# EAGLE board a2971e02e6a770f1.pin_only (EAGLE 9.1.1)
REV: C

Size 60 x 60 mm. Coordinates in mm from the lower left corner, seen from the top.
Outline: 60,0 0,0 0,60 60,60 60,0
Copper layers (1*16): Top 0.035mm / dielectric 1.5mm / Bottom 0.035mm
Design rules "adafruit 88 *": minimum track width 8mil, minimum drill 15.5mil, track to track 8mil, track to pad 8mil, pad to pad 8mil, via to via 8mil, smd to smd 8mil, copper to edge 10mil, drill to drill 8mil, minimum pad ring 10mil, minimum via ring 8mil, stop-mask expansion 2mil, vias tented up to drill 20mil, thermal gap 10mil
Net classes: 1 power: width 0.406 mm; 2 gnd: width 0.254 mm
Holes 2.8 mm at 2.03,44.97 28.03,44.97 32.03,44.97 58.03,44.97 2.03,14.97 28.03,14.97 32.03,14.97 58.03,14.97
Holes 2 mm at 15.03,44.97 45.03,44.97 15.03,14.97 45.03,14.97
Holes 1 mm at 1.33,58.67 58.73,58.67 1.33,1.27 58.73,1.27

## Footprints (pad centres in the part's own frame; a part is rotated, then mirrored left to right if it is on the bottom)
0805-NO = smd 1.24 x 1.5: 1 -0.95,0; 2 0.95,0
0603-NO = smd 1.075 x 1: 1 -0.85,0; 2 0.85,0
SOD-323 = smd 1.35 x 0.8: A 1.27,0; C -1.27,0
FIDUCIAL_1MM = smd 1 x 1: 1 0,0
QFN24_4MM = smd 0.8 x 0.28: 1 -2,1.25; 2 -2,0.75; 3 -2,0.25; 4 -2,-0.25; 5 -2,-0.75; 6 -2,-1.25; 13 2,-1.25; 14 2,-0.75; 15 2,-0.25; 16 2,0.25; 17 2,0.75; 18 2,1.25 | smd 0.28 x 0.8: 7 -1.25,-2; 8 -0.75,-2; 9 -0.25,-2; 10 0.25,-2; 11 0.75,-2; 12 1.25,-2; 19 1.25,2; 20 0.75,2; 21 0.25,2; 22 -0.25,2; 23 -0.75,2; 24 -1.25,2 | smd 1.778 x 1.778: THERM 0,0
SOT23-5 = smd 0.69 x 0.99: 1 -0.95,-1.29; 2 0,-1.29; 3 0.95,-1.29; 4 0.95,1.3; 5 -0.95,1.3
5P_EDGECONNECT = smd 1.27 x 5.08: 1 -5.08,0; 2 -2.54,0; 3 0,0; 4 2.54,0; 5 5.08,0
LED3535 = smd 1 x 0.85: 1 -1.75,0.875; 2 -1.75,-0.875; 3 1.75,-0.875; 4 1.75,0.875
SOT23-WIDE = smd 1 x 1.2: 1 -0.95,-1; 2 0.95,-1; 3 0,1
SOLDERJUMPER_ARROW_NOPASTE = smd 0.762 x 1.524: 1 -1.016,0; 2 1.016,0
SOLDERJUMPER_2WAY_OPEN_NOPASTE = smd 1.168 x 1.6: 1 -1.397,0; 2 0,0; 3 1.397,0
TESTPOINT_SMT = smd 4.7 x 3.4: P$1 0,0
TESTPOINT_ROUND_2MM = smd 2 x 2: P$1 0,0
TESTPOINT_ROUND_1.5MM = smd 1.5 x 1.5: P$1 0,0
SOT23-5' = smd 0.55 x 1.2: 1 -0.95,-1.3; 2 0,-1.3; 3 0.95,-1.3; 4 0.95,1.3; 5 -0.95,1.3
MOUNTINGHOLE_2.5_PLATED = drill 2.5 pad 3.2: P$1 0,0
ELAST_PAD_SQUARE_10MM_4X4WIDE = smd 1.45 x 0.635: P$1 -3.4,0 | smd 0.305 x 0.61: P$2 4,0
JSTPH4 = smd 1 x 4.6: 1 -3,-3.7; 2 -1,-3.7; 3 1,-3.7; 4 3,-3.7 | smd 1.7 x 3.4: NC1 -5.7,1.5; NC2 5.7,1.5

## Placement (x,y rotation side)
C1  10u  [0805-NO]  52.13,26.04 0 top
C2  10u  [0805-NO]  8.69,26.16 270 top
C3  10u  [0805-NO]  31.55,6.1 0 top
C4  10u  [0805-NO]  33.84,52.7 90 top
C7  1uF  [0603-NO]  25.58,47.85 0 top
C8  10µF  [0805-NO]  24.63,45.22 270 top
D1  1N4148  [SOD-323]  37.59,48.95 180 top
D2  1N4148  [SOD-323]  22.59,48.95 0 top
D3  1N4148  [SOD-323]  9.66,50.09 0 top
D4  1N4148  [SOD-323]  52.62,40.96 180 top
D5  1N4148  [SOD-323]  37.61,40.96 180 top
D6  1N4148  [SOD-323]  22.69,40.96 0 top
D7  1N4148  [SOD-323]  7.92,40.71 0 top
D8  1N4148  [SOD-323]  52.68,18.97 180 top
D9  1N4148  [SOD-323]  52.58,48.94 180 top
D10  1N4148  [SOD-323]  37.7,18.84 180 top
D11  1N4148  [SOD-323]  14.06,18.86 180 top
D12  1N4148  [SOD-323]  7.4,18.83 0 top
D13  1N4148  [SOD-323]  52.48,11.01 180 top
D14  1N4148  [SOD-323]  37.62,11.01 180 top
D15  1N4148  [SOD-323]  13.11,10.98 180 top
D16  1N4148  [SOD-323]  7.45,11.02 0 top
FID1  FIDUCIAL_1MM  [FIDUCIAL_1MM]  10.23,14.05 0 top
FID2  FIDUCIAL_1MM  [FIDUCIAL_1MM]  58.48,11.68 0 top
FID3  FIDUCIAL_1MM  [FIDUCIAL_1MM]  56.25,54.98 0 top
FID4  FIDUCIAL_1MM  [FIDUCIAL_1MM]  51.36,46.1 0 bottom
FID5  FIDUCIAL_1MM  [FIDUCIAL_1MM]  44.76,7.11 0 bottom
FID6  FIDUCIAL_1MM  [FIDUCIAL_1MM]  7.93,15.75 0 bottom
IC2  ATSAMD09D14A-MU  [QFN24_4MM]  38.96,31.87 270 top
IC3  74AHCT1G125DBV  [SOT23-5]  47.3,50.29 90 top
JP1  [5P_EDGECONNECT]  2.6,29.97 90 top
JP2  [5P_EDGECONNECT]  57.46,29.97 90 top
JP3  [5P_EDGECONNECT]  30.03,2.54 180 top
JP4  [5P_EDGECONNECT]  30.03,57.4 180 top
LED1  WS2812B3535  [LED3535]  52.53,52.47 270 bottom
LED2  WS2812B3535  [LED3535]  37.53,52.47 270 bottom
LED3  WS2812B3535  [LED3535]  22.53,52.47 270 bottom
LED4  WS2812B3535  [LED3535]  7.53,52.47 270 bottom
LED5  WS2812B3535  [LED3535]  52.53,37.47 270 bottom
LED6  WS2812B3535  [LED3535]  37.53,37.47 270 bottom
LED7  WS2812B3535  [LED3535]  22.53,37.47 270 bottom
LED8  WS2812B3535  [LED3535]  7.53,37.47 270 bottom
LED9  WS2812B3535  [LED3535]  52.53,22.47 270 bottom
LED10  WS2812B3535  [LED3535]  37.53,22.47 270 bottom
LED11  WS2812B3535  [LED3535]  7.53,22.47 270 bottom
LED12  WS2812B3535  [LED3535]  22.53,22.47 270 bottom
LED13  WS2812B3535  [LED3535]  52.53,7.47 270 bottom
LED14  WS2812B3535  [LED3535]  37.53,7.47 270 bottom
LED15  WS2812B3535  [LED3535]  22.53,7.47 270 bottom
LED16  WS2812B3535  [LED3535]  7.53,7.47 270 bottom
Q1  BSS138  [SOT23-WIDE]  7.93,46.1 90 top
Q2  BSS138  [SOT23-WIDE]  11.74,46.1 270 top
R3  10k  [0603-NO]  37.8,45.47 90 top
R4  10K  [0603-NO]  11.36,43.43 180 top
R5  10K  [0603-NO]  9.71,48.51 0 top
R6  10K  [0603-NO]  14.41,47.75 0 top
R7  10K  [0603-NO]  52.81,33.48 0 top
R8  10K  [0603-NO]  11.61,41.4 0 top
SJ1  [SOLDERJUMPER_ARROW_NOPASTE]  32.23,27.71 180 top
SJ2  [SOLDERJUMPER_ARROW_NOPASTE]  32.23,29.96 180 top
SJ3  [SOLDERJUMPER_ARROW_NOPASTE]  32.23,32.2 180 top
SJ4  [SOLDERJUMPER_2WAY_OPEN_NOPASTE]  17.84,45.72 270 top
SJ8  [SOLDERJUMPER_ARROW_NOPASTE]  37.29,26.72 270 top
SJ9  [SOLDERJUMPER_ARROW_NOPASTE]  35.17,26.72 270 top
TP1  [TESTPOINT_SMT]  58.22,29.97 90 bottom
TP2  [TESTPOINT_SMT]  29.77,1.78 0 bottom
TP3  [TESTPOINT_SMT]  30.03,58.17 0 bottom
TP4  [TESTPOINT_SMT]  1.71,29.97 90 bottom
TP5  [TESTPOINT_ROUND_2MM]  48.64,30.37 0 top
TP6  [TESTPOINT_ROUND_2MM]  50.04,32.61 0 top
TP7  [TESTPOINT_ROUND_1.5MM]  40.7,27.05 0 top
TP8  [TESTPOINT_ROUND_1.5MM]  50.6,43.43 0 top
TP9  [TESTPOINT_ROUND_1.5MM]  20.63,19.43 0 top
TP10  [TESTPOINT_ROUND_1.5MM]  19.49,12.7 0 top
TP11  [TESTPOINT_ROUND_1.5MM]  47.55,35.69 0 top
TP12  [TESTPOINT_ROUND_1.5MM]  35.87,35.05 0 top
TP13  [TESTPOINT_ROUND_1.5MM]  30.79,36.32 0 top
TP14  [TESTPOINT_ROUND_1.5MM]  11.61,34.04 0 top
TP24  [TESTPOINT_ROUND_1.5MM]  12.12,51.56 0 top
U2  AP2112-3.3  [SOT23-5']  21.53,45.22 270 top
U$1  MOUNTINGHOLE2.5  [MOUNTINGHOLE_2.5_PLATED]  45.01,29.97 0 bottom
U$2  MOUNTINGHOLE2.5  [MOUNTINGHOLE_2.5_PLATED]  15.04,29.97 0 bottom
U$3  [ADAFRUIT_TEXT_20MM]  38.28,0.38 0 top
U$4  ELAST_10X10  [ELAST_PAD_SQUARE_10MM_4X4WIDE]  52.53,52.47 180 bottom
U$5  ELAST_10X10  [ELAST_PAD_SQUARE_10MM_4X4WIDE]  37.53,52.47 180 bottom
U$6  ELAST_10X10  [ELAST_PAD_SQUARE_10MM_4X4WIDE]  22.53,52.47 0 bottom
U$7  ELAST_10X10  [ELAST_PAD_SQUARE_10MM_4X4WIDE]  7.53,52.47 0 bottom
U$8  ELAST_10X10  [ELAST_PAD_SQUARE_10MM_4X4WIDE]  52.53,37.47 180 bottom
U$9  ELAST_10X10  [ELAST_PAD_SQUARE_10MM_4X4WIDE]  37.53,37.47 180 bottom
U$10  ELAST_10X10  [ELAST_PAD_SQUARE_10MM_4X4WIDE]  22.53,37.47 0 bottom
U$11  ELAST_10X10  [ELAST_PAD_SQUARE_10MM_4X4WIDE]  7.53,37.47 0 bottom
U$12  ELAST_10X10  [ELAST_PAD_SQUARE_10MM_4X4WIDE]  52.53,22.47 180 bottom
U$14  [SEESAW_LOGO]  2.09,1.52 0 top
U$19  [PCBFEAT-REV-040]  53.9,14.61 0 top
U$23  ELAST_10X10  [ELAST_PAD_SQUARE_10MM_4X4WIDE]  37.53,22.47 180 bottom
U$24  ELAST_10X10  [ELAST_PAD_SQUARE_10MM_4X4WIDE]  7.53,22.47 0 bottom
U$25  ELAST_10X10  [ELAST_PAD_SQUARE_10MM_4X4WIDE]  22.53,22.47 0 bottom
U$26  ELAST_10X10  [ELAST_PAD_SQUARE_10MM_4X4WIDE]  52.53,7.47 180 bottom
U$27  ELAST_10X10  [ELAST_PAD_SQUARE_10MM_4X4WIDE]  37.53,7.47 180 bottom
U$28  ELAST_10X10  [ELAST_PAD_SQUARE_10MM_4X4WIDE]  22.53,7.47 0 bottom
U$29  ELAST_10X10  [ELAST_PAD_SQUARE_10MM_4X4WIDE]  7.53,7.47 0 bottom
X2  STEMMA_I2C_RASMT  [JSTPH4]  23.55,29.21 180 top

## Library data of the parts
C1-C4 C7 C8 D1-D16 IC2 JP1-JP4 LED1-LED16 Q1 Q2 R3-R8 SJ4 TP1-TP14 TP24 U2 U$3-U$12 U$19 U$23-U$29 X2 = microbuilder
FID1-FID6 SJ1-SJ3 SJ8 SJ9 U$1 U$2 = microbuilder; BOM: EXCLUDE
IC3 = 74xx-little-us
U$14 = silks

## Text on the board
tPlace: 4x4 Elastomer / Buttons+LEDs | SDA | SCL | GND | VIN | INT | Tile together w/ / unique addrs | 3V | Vi2c | Vin | Adafruit NeoTrellis 4x4 | SDA | SDA | SCL | SDA | Vin | GND | GND | SCL | SCL | A4 | GND | GND | A3 | VIN | VIN | A2 | INT | INT | A1 | A0 | GND | VIN | SDA | SCL | INT
bPlace: 4 | 3 | 2 | 1 | 8 | 7 | 6 | 5 | 12 | 11 | 10 | 9 | 16 | 15 | 13 | 14

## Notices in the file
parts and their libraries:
microbuilder: This work is placed in the public domain, and may be freely used for commercial and non-commercial work with the following conditions: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
